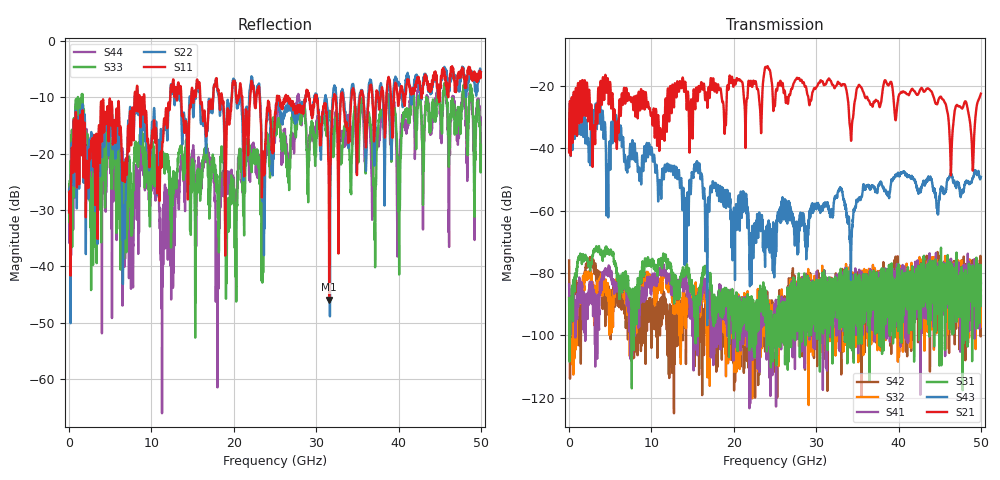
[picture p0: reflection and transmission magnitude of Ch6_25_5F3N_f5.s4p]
!Agilent Technologies,N5247A,US51170199,A.09.90.13
!Agilent N5247A: A.09.90.13
!Date: Wednesday, December 16, 2015 09:52:20
!Correction: S11(Full 4 Port(1,2,3,4))
!S12(Full 4 Port(1,2,3,4))
!S13(Full 4 Port(1,2,3,4))
!S14(Full 4 Port(1,2,3,4))
!S21(Full 4 Port(1,2,3,4))
!S22(Full 4 Port(1,2,3,4))
!S23(Full 4 Port(1,2,3,4))
!S24(Full 4 Port(1,2,3,4))
!S31(Full 4 Port(1,2,3,4))
!S32(Full 4 Port(1,2,3,4))
!S33(Full 4 Port(1,2,3,4))
!S34(Full 4 Port(1,2,3,4))
!S41(Full 4 Port(1,2,3,4))
!S42(Full 4 Port(1,2,3,4))
!S43(Full 4 Port(1,2,3,4))
!S44(Full 4 Port(1,2,3,4))
!S4P File: Measurements: <S11,S12,S13,S14>,
!<S21,S22,S23,S24>,
!<S31,S32,S33,S34>,
!<S41,S42,S43,S44>:
# Hz S  dB  R 50
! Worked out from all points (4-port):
!   3201 points, 10 MHz to 50 GHz, reference 50 ohm
!   strongest paths, dB at 10 MHz, 12.51 GHz, 25 GHz, 37.5 GHz, 50 GHz:
!     S21: -41.3, -21.5, -26.2, -24.9, -22.5
!     S43: -40.8, -45.8, -75.6, -52.6, -49.2
!     S31: -88.0, -83.6, -94.5, -84.1, -83.4
!     S41: -83.6, -82.9, -95.9, -96.7, -83.0
!     S32: -87.8, -88.2, -92.6, -96.4, -85.5
!     S42: -76.0, -102.3, -95.5, -87.4, -87.4
!   lowest |S11| = -45.9 dB at 31.58 GHz (marker M1), VSWR 1.01, Z = 49.5 - j0.0505 ohm
!   |S11| at or under -10 dB: start of sweep to 7.958 GHz; 9.141 GHz to 12.29 GHz (3.144 GHz wide, 29.4 % of centre); 26.6 GHz to 28.71 GHz (2.113 GHz wide, 7.64 % of centre)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
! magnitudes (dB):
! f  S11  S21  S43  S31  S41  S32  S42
! 10 MHz  -30.4  -41.3  -40.8  -88.0  -83.6  -87.8  -76.0
! 12.54 GHz  -8.5  -19.9  -46.3  -83.1  -84.6  -87.8  -90.7
! 22.11 GHz  -7.5  -18.7  -78.0  -99.2  -93.6  -92.1  -93.1
! 23.61 GHz  -20.9  -17.4  -69.9  -90.3  -96.8  -90.0  -95.1
! 31.58 GHz  -45.9  -17.7  -60.5  -94.5  -83.3  -85.9  -95.6
! 46.38 GHz  -4.6  -47.8  -48.2  -79.8  -75.4  -77.1  -84.8
! 50 GHz  -5.6  -22.5  -49.2  -83.4  -83.0  -85.5  -87.4
